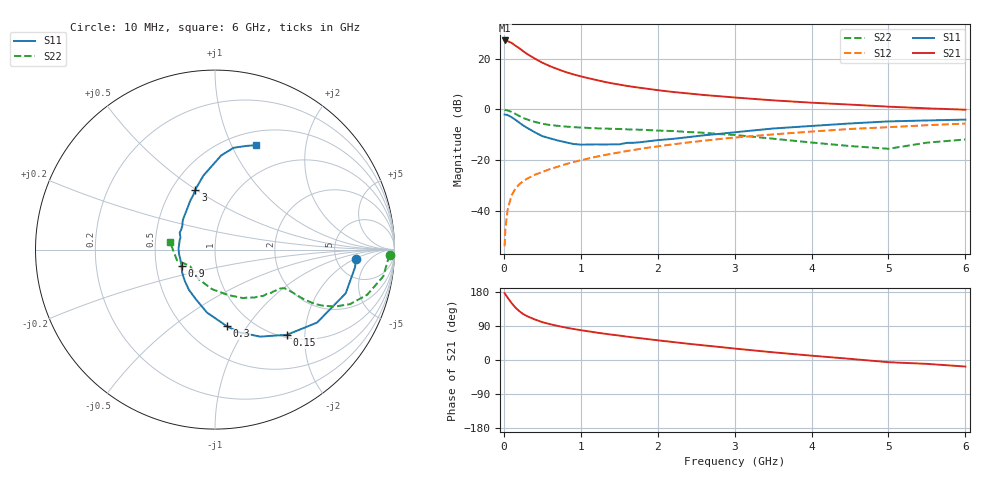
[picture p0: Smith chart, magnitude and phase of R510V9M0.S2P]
! SIEMENS Small Signal Semiconductors
! BFR183
! Si NPN RF Bipolar Junction Transistor in SOT23
! VCE = 10 V  IC = 9 mA
! Common Emitter S-Parameters:  May  1996
# GHz  S  MA  R  50
!  f  S11  S21  S12  S22
! GHz  MAG  ANG  MAG  ANG  MAG  ANG  MAG  ANG
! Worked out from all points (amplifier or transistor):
!   36 points, 10 MHz to 6 GHz, reference 50 ohm
!   highest |S21| = 27.1 dB at 10 MHz (marker M1)
!   |S21| within 3 dB of that: start of sweep to 197.5 MHz
!   unconditionally stable (mu >= 1): 871.3 MHz to 2.69 GHz
!   at 250 MHz: K = 0.57, MSG = 25.7 dB, |S12| = -28.4 dB
!   at 1.4 GHz: K = 1.05, MAG = 12.5 dB, |S12| = -17.6 dB
!   at 6 GHz: K = 0.88, MSG = 2.7 dB, |S12| = -5.6 dB
!   S11 on the Smith chart (normalised r, x): 10 MHz: 7.78, -2.13; 150 MHz: 1.05, -1.62; 300 MHz: 0.77, -0.81; 900 MHz: 0.68, -0.13; 3 GHz: 0.65, +0.50; 6 GHz: 0.65, +1.25
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0.01  0.7867 -3.8  22.74 176.3  0.002 79.6  0.9736 -1.8
0.02  0.7865 -7.2  22.28 173.1  0.0044 84.7  0.9649 -3.6
0.05  0.7679 -18.5  22.02 164.3  0.0106 80.2  0.9495 -9.0
0.1  0.6989 -35.6  20.39 150.5  0.0199 73.8  0.8838 -16.6
0.15  0.6212 -49.8  17.97 138.4  0.0273 67.5  0.811 -22.0
0.2  0.5466 -62.5  16.01 129.1  0.0331 64.6  0.7399 -25.4
0.25  0.4818 -73.4  14.04 121.5  0.0382 63.0  0.6759 -27.5
0.3  0.4327 -81.1  12.38 115.9  0.0426 62.5  0.6315 -28.6
0.4  0.3538 -97.2  10.03 107.2  0.0509 61.5  0.5653 -29.2
0.5  0.2958 -111.3  8.287 99.9  0.058 62.5  0.5175 -29.1
0.6  0.2672 -122.9  7.078 94.6  0.0663 62.8  0.4898 -28.9
0.7  0.2428 -133.8  6.177 89.9  0.0737 63.3  0.4723 -28.9
0.9  0.2074 -154.0  4.897 82.0  0.0906 63.7  0.4453 -29.0
1.1  0.2017 -172.5  4.095 75.6  0.1071 64.1  0.429 -30.3
1.3  0.2018 172.2  3.497 69.7  0.1244 63.4  0.417 -31.8
1.6  0.2178 154.5  2.887 61.7  0.1502 61.8  0.4022 -35.2
2.2  0.2611 129.1  2.192 47.4  0.2038 57.5  0.3726 -43.8
3  0.3519 108.1  1.707 30.2  0.2768 49.5  0.3119 -60.0
3.5  0.4176 98.9  1.5 20.3  0.3197 43.5  0.263 -74.1
4.5  0.5253 86.3  1.237 3.1  0.409 31.8  0.1885 -118.9
5.5  0.602 73.5  1.044 -10.2  0.4855 20.5  0.2199 -164.2
6  0.6256 68.5  0.981 -17.3  0.5228 13.0  0.2536 170.8
